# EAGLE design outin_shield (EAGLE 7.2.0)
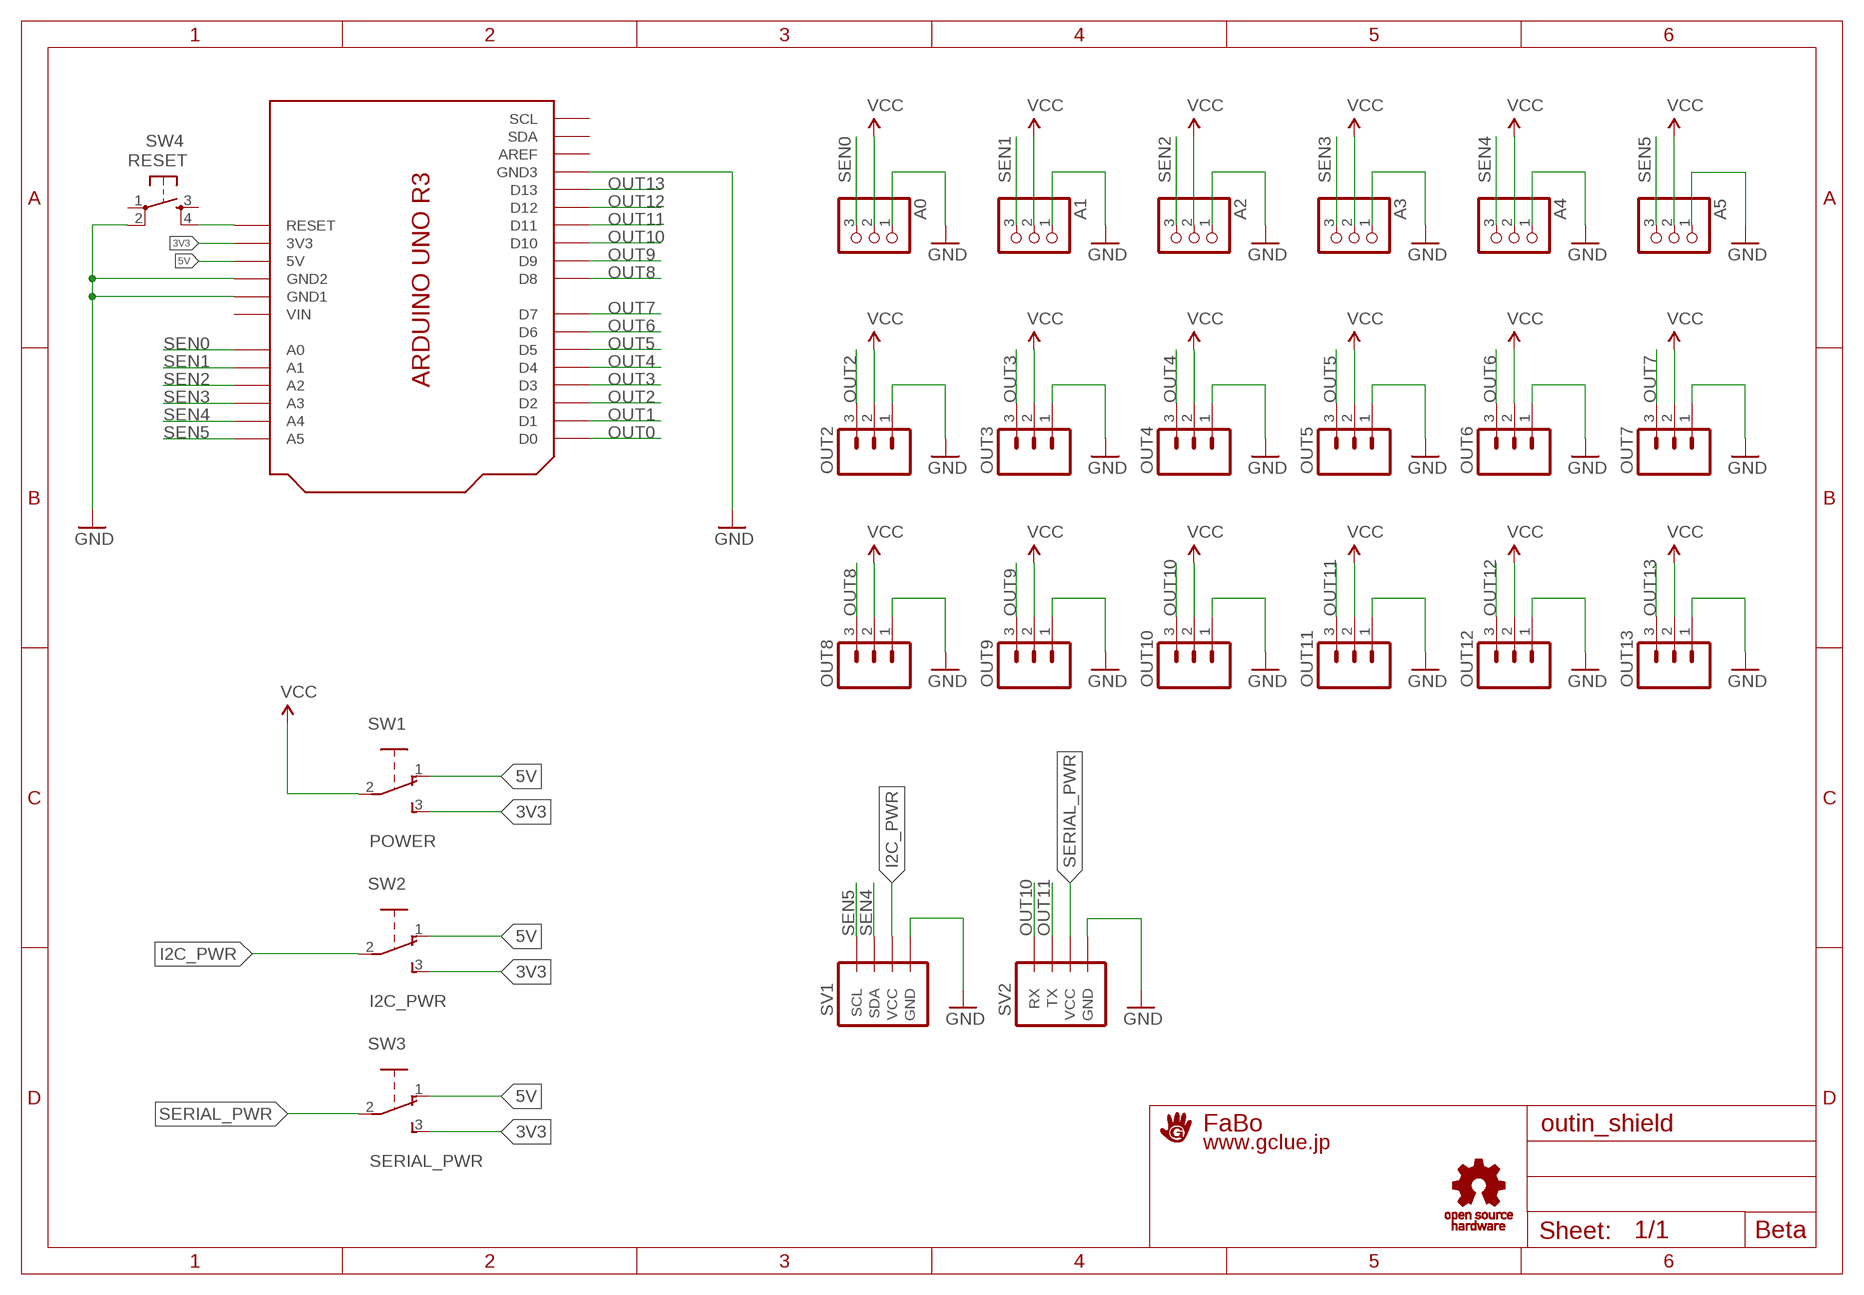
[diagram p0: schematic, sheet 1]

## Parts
A0  PINHD-1X3  [1X03]
A1  PINHD-1X3  [1X03]
A2  PINHD-1X3  [1X03]
A3  PINHD-1X3  [1X03]
A4  PINHD-1X3  [1X03]
A5  PINHD-1X3  [1X03]
OUT2  M03PTH  [1X03]
OUT3  M03PTH  [1X03]
OUT4  M03PTH  [1X03]
OUT5  M03PTH  [1X03]
OUT6  M03PTH  [1X03]
OUT7  M03PTH  [1X03]
OUT8  M03PTH  [1X03]
OUT9  M03PTH  [1X03]
OUT10  M03PTH  [1X03]
OUT11  M03PTH  [1X03]
OUT12  M03PTH  [1X03]
OUT13  M03PTH  [1X03]
SV1  BRICK_I2C_CONNECTOR  [BRICK_I2C_CONNECTOR]
SV2  BRICK_SERIAL_CONNECTOR  [BRICK_SERIAL_CONNECTOR]
SW1  POWER  SWITCH-SLIDE-EG1218  [EG1218]
SW2  I2C_PWR  SWITCH-SLIDE-EG1218  [EG1218]
SW3  SERIAL_PWR  SWITCH-SLIDE-EG1218  [EG1218]
SW4  RESET  TAC_SWITCHPTH  [TACTILE-PTH]
U1  OUTIN_SHIELD  [ARDUINO_UNO_R3_OUTIN]
U$2  LOGO_GCLUE-M  [LOGO_GCLUE_M]
U$3  LOGO_OSHW_T-M  [LOGO_OSHW_T_M]

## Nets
3V3 [POWER]: SW1.3 SW2.3 SW3.3 U1.3V3
5V [POWER]: SW1.1 SW2.1 SW3.1 U1.5V
GND [POWER]: A0.1 A1.1 A2.1 A3.1 A4.1 A5.1 OUT2.1 OUT3.1 OUT4.1 OUT5.1 OUT6.1 OUT7.1 OUT8.1 OUT9.1 OUT10.1 OUT11.1 OUT12.1 OUT13.1 SV1.GND SV2.GND SW4.2 U1.GND1 U1.GND2 U1.GND3
I2C_PWR [POWER]: SV1.VCC SW2.2
OUT0: U1.D0
OUT1: U1.D1
OUT2: OUT2.3 U1.D2
OUT3: OUT3.3 U1.D3
OUT4: OUT4.3 U1.D4
OUT5: OUT5.3 U1.D5
OUT6: OUT6.3 U1.D6
OUT7: OUT7.3 U1.D7
OUT8: OUT8.3 U1.D8
OUT9: OUT9.3 U1.D9
OUT10: OUT10.3 SV2.RX U1.D10
OUT11: OUT11.3 SV2.TX U1.D11
OUT12: OUT12.3 U1.D12
OUT13: OUT13.3 U1.D13
RESET: SW4.4 U1.RESET
SEN0: A0.3 U1.A0
SEN1: A1.3 U1.A1
SEN2: A2.3 U1.A2
SEN3: A3.3 U1.A3
SEN4: A4.3 SV1.SDA U1.A4
SEN5: A5.3 SV1.SCL U1.A5
SERIAL_PWR [POWER]: SV2.VCC SW3.2
VCC [POWER]: A0.2 A1.2 A2.2 A3.2 A4.2 A5.2 OUT2.2 OUT3.2 OUT4.2 OUT5.2 OUT6.2 OUT7.2 OUT8.2 OUT9.2 OUT10.2 OUT11.2 OUT12.2 OUT13.2 SW1.2
Unconnected: SW4.1 SW4.3 U1.AREF U1.SCL U1.SDA

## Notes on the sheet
- RESET
- Beta

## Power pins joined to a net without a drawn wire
VIN: U1.VIN

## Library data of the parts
A0 A1-A5 = adafruit:PINHD-1X3: PIN HEADER
OUT2-OUT13 = SparkFun:M03: Header 3 Standard 3-pin 0.1" header. Use with straight break away headers (SKU : PRT-00116), right angle break away headers (PRT-00553), swiss pins (PRT-00743), machine pins (PRT-00117), and female headers (PRT-00115). Molex polarized connector foot print use with SKU : PRT-08232 with associated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
SV1 = Gclue:BRICK_I2C_CONNECTOR: Brick Connector female for OUT/IN Shield
SV2 = Gclue:BRICK_SERIAL_CONNECTOR
SW1-SW3 = Gclue:SWITCH-SLIDE
SW4 = SparkFun-3-2-07:TAC_SWITCH: Momentary Switch Button commonly used for reset or general input. Spark Fun Electronics SKU : Comp-PBS
U1 = Gclue:OUTIN_SHIELD
U$2 = Gclue:LOGO_GCLUE
U$3 = Gclue:LOGO_OSHW_T

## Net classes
1 POWER: width 0.406 mm

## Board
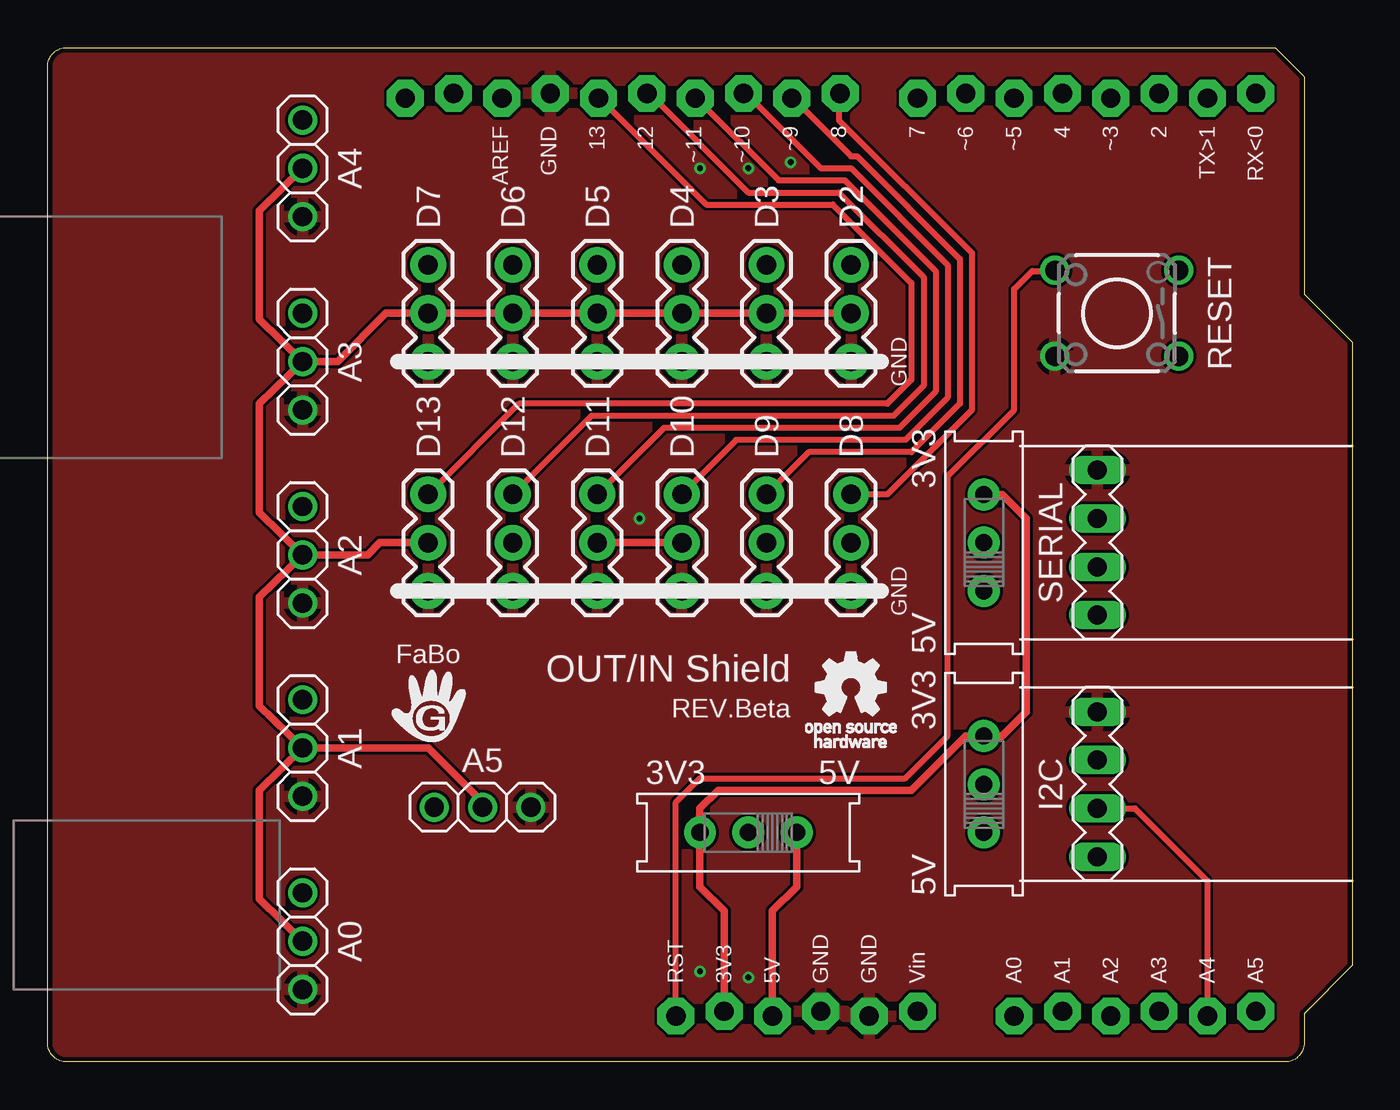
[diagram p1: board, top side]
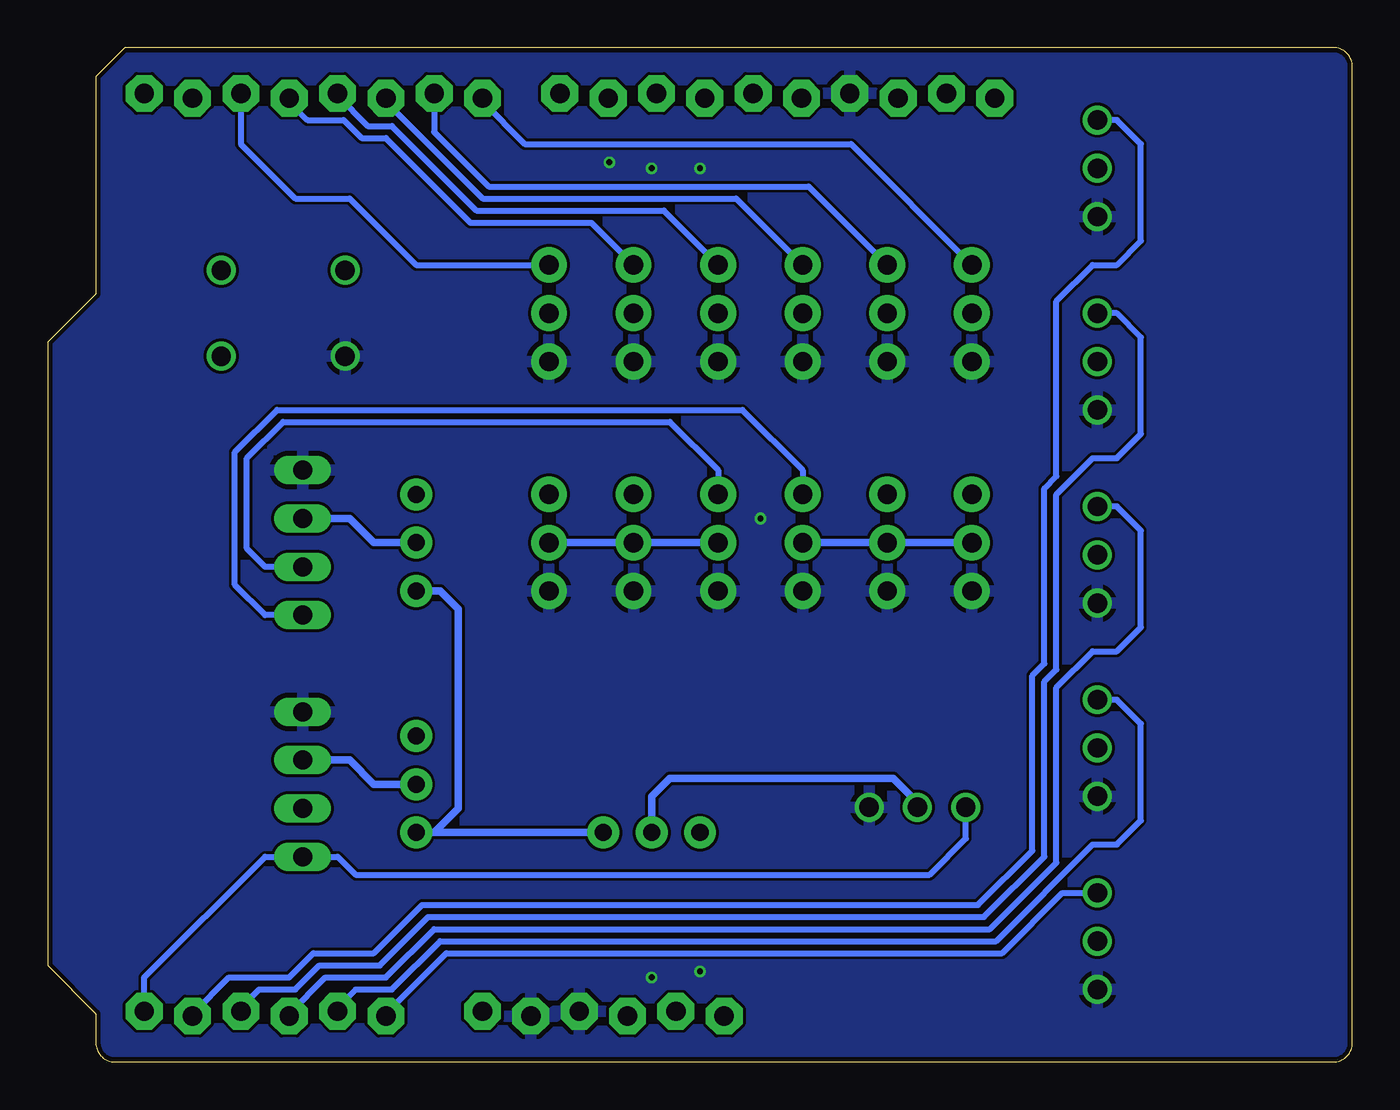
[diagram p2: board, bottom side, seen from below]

Size 68.58 x 53.34 mm. Coordinates in mm from the lower left corner, seen from the top.
Copper layers (1*16): Top 0.035mm / dielectric 1.5mm / Bottom 0.035mm
Design rules "Elecrow_2-layer_eagle_rule": minimum track width 6mil, minimum drill 12mil, track to track 6mil, track to pad 6mil, pad to pad 6mil, via to via 6mil, smd to smd 0mil, copper to edge 10mil, drill to drill 10mil, minimum pad ring 10mil, minimum via ring 6mil, stop-mask expansion 2mil, vias tented up to drill 100mil, thermal gap 10mil

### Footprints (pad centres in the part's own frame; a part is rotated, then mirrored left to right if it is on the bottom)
1X03 = drill 1.016: 1 -2.54,0; 2 0,0; 3 2.54,0
1X03' = drill 1.016 pad 1.88: 1 0,0; 2 2.54,0; 3 5.08,0
BRICK_I2C_CONNECTOR = drill 1 long: GND -3.81,0; SCL 3.81,0; SDA 1.27,0; VCC -1.27,0
BRICK_SERIAL_CONNECTOR = drill 1 long: GND -3.81,0; RX 1.27,0; TX 3.81,0; VCC -1.27,0
EG1218 = drill 0.9 pad 1.676: 1 -2.54,0; 2 0,0; 3 2.54,0
TACTILE-PTH = drill 1.016: 1 -3.251,2.261; 2 3.251,2.261; 3 -3.251,-2.261; 4 3.251,-2.261
ARDUINO_UNO_R3_OUTIN = drill 1.016 pad 1.93 octagon: 3V3 35.56,2.667; 5V 38.1,2.413; A0 50.8,2.413; A1 53.34,2.667; A2 55.88,2.413; A3 58.42,2.667; A4 60.96,2.413; A5 63.5,2.667; AREF 23.876,50.673; D0 63.5,50.927; D1 60.96,50.673; D2 58.42,50.927; D3 55.88,50.673; D4 53.34,50.927; D5 50.8,50.673; D6 48.26,50.927; D7 45.72,50.673; D8 41.656,50.927; D9 39.116,50.673; D10 36.576,50.927; D11 34.036,50.673; D12 31.496,50.927; D13 28.956,50.673; GND1 43.18,2.413; GND2 40.64,2.667; GND3 26.416,50.927; RESET 33.02,2.413; SCL 18.796,50.673; SDA 21.336,50.927; VIN 45.72,2.667

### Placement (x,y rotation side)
A0  13.4,6.35 90 top
A1  13.4,16.51 90 top
A2  13.4,26.67 90 top
A3  13.4,36.83 90 top
A4  13.4,46.99 90 top
A5  22.86,13.4 180 top
OUT2  [1X03']  42.23,36.83 90 top
OUT3  [1X03']  37.78,36.83 90 top
OUT4  [1X03']  33.34,36.83 90 top
OUT5  [1X03']  28.89,36.83 90 top
OUT6  [1X03']  24.45,36.83 90 top
OUT7  [1X03']  20,36.83 90 top
OUT8  [1X03']  42.23,24.77 90 top
OUT9  [1X03']  37.78,24.77 90 top
OUT10  [1X03']  33.34,24.77 90 top
OUT11  [1X03']  28.89,24.77 90 top
OUT12  [1X03']  24.45,24.77 90 top
OUT13  [1X03']  20,24.77 90 top
SV1  55.18,14.61 270 top
SV2  55.18,27.3 270 top
SW1  36.83,12.06 180 top
SW2  49.21,14.61 90 top
SW3  49.21,27.3 90 top
SW4  56.2,39.37 180 top
U1  0,0 0 top
U$2  20,18.73 0 top
U$3  42.23,19.68 0 top

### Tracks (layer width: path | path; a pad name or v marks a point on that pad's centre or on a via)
3V3
  Top 0.406: U1.3V3 35.56,7.94 34.29,9.21 SW1.3 34.29,13.34 35.24,14.29 45.4,14.29 48.26,17.14 SW2.3 50.16,17.14 51.44,18.41 51.44,28.57 50.16,29.84 SW3.3
5V
  Top 0.406: U1.5V 38.1,7.94 39.37,9.21 SW1.1
  Bottom 0.406: SW1.1 48.26,12.06 | SW2.1 48.26,12.06 | 48.26,12.06 46.99,13.34 46.99,23.81 47.94,24.77 SW3.1
GND  (via drill 0.3)
  other vias: 36.83,4.45 34.29,4.76 31.11,28.57 34.29,46.99 36.83,46.99 39.05,47.31
  pour Bottom: -7.3,54.29 69.53,54.29 69.53,-0.95 -7.3,-0.95
  pour Top: -7.3,54.29 69.53,54.29 69.53,-0.95 -7.3,-0.95
I2C_PWR
  Bottom 0.406: SW2.2 51.44,14.61 52.7,15.88 SV1.VCC
OUT2
  Bottom 0.305: U1.D2 58.42,48.26 55.56,45.4 52.7,45.4 49.21,41.91 OUT2.3
OUT3
  Bottom 0.305: U1.D3 55.88,50.48 54.93,49.53 53.02,49.53 52.07,48.58 50.8,48.58 46.35,44.13 40.01,44.13 OUT3.3
OUT4
  Bottom 0.305: U1.D4 53.34,50.8 51.75,49.21 50.48,49.21 46.04,44.77 36.2,44.77 OUT4.3
OUT5
  Bottom 0.305: U1.D5 50.8,50.48 45.72,45.4 32.38,45.4 OUT5.3
OUT6
  Bottom 0.305: U1.D6 48.26,48.9 45.4,46.04 28.57,46.04 OUT6.3
OUT7
  Bottom 0.305: U1.D7 45.72,50.48 43.5,48.26 26.35,48.26 OUT7.3
OUT8
  Top 0.305: U1.D8 41.59,50.8 41.59,49.53 48.58,42.55 48.58,34.29 44.13,29.84 OUT8.3
OUT9
  Top 0.305: U1.D9 39.37,50.48 42.23,47.62 42.55,47.62 47.94,42.23 47.94,34.61 45.4,32.07 40.01,32.07 OUT9.3
OUT10
  Top 0.305: U1.D10 36.83,50.8 40.64,46.99 42.23,46.99 47.31,41.91 47.31,34.92 45.09,32.7 36.2,32.7 OUT10.3
  Bottom 0.305: SV2.RX 57.15,26.04 58.1,26.99 58.1,31.75 56.2,33.66 35.88,33.66 33.34,31.11 OUT10.3
OUT11
  Top 0.305: U1.D11 34.29,50.48 38.42,46.35 41.91,46.35 46.67,41.59 46.67,35.24 44.77,33.34 32.38,33.34 OUT11.3
  Bottom 0.305: SV2.TX 57.15,23.5 58.74,25.08 58.74,32.07 56.52,34.29 32.07,34.29 28.89,31.11 OUT11.3
OUT12
  Top 0.305: U1.D12 31.75,50.8 36.83,45.72 41.59,45.72 46.04,41.27 46.04,35.56 44.45,33.97 28.57,33.97 OUT12.3
OUT13
  Top 0.305: U1.D13 29.21,50.48 34.61,45.09 41.27,45.09 45.4,40.96 45.4,35.88 44.13,34.61 24.77,34.61 OUT13.3
RESET
  Top 0.305: U1.RESET 33.02,13.65 34.29,14.92 45.09,14.92 47.31,17.14 47.31,30.8 50.8,34.29 50.8,40.64 51.75,41.59 52.7,41.59 SW4.4
SEN0
  Bottom 0.305: U1.A0 50.8,2.54 47.62,5.71 18.41,5.71 15.24,8.89 A0.3
SEN1
  Bottom 0.305: U1.A1 53.34,2.86 52.39,3.81 50.48,3.81 47.94,6.35 18.73,6.35 13.65,11.43 12.38,11.43 11.11,12.7 11.11,17.78 12.38,19.05 A1.3
SEN2
  Bottom 0.305: U1.A2 55.88,2.54 53.98,4.45 50.8,4.45 48.26,6.99 19.05,6.99 15.56,10.48 15.56,19.68 13.65,21.59 12.38,21.59 11.11,22.86 11.11,27.94 12.38,29.21 A2.3
SEN3
  Bottom 0.305: U1.A3 58.42,2.86 57.47,3.81 55.56,3.81 54.29,5.08 51.12,5.08 48.58,7.62 19.37,7.62 16.19,10.79 16.19,20 15.56,20.64 15.56,29.84 13.65,31.75 12.38,31.75 11.11,33.02 11.11,38.1 12.38,39.37 A3.3
SEN4
  Top 0.305: SV1.SDA 57.15,13.34 60.96,9.53 U1.A4
  Bottom 0.305: U1.A4 60.96,2.54 59.05,4.45 55.88,4.45 54.61,5.71 51.44,5.71 48.9,8.26 19.68,8.26 16.83,11.11 16.83,20.32 16.19,20.95 16.19,30.16 15.56,30.8 15.56,40.01 13.65,41.91 12.38,41.91 11.11,43.18 11.11,48.26 12.38,49.53 A4.3
SEN5
  Bottom 0.305: U1.A5 63.5,4.45 57.15,10.79 SV1.SCL 53.34,10.79 52.39,9.84 22.23,9.84 20.32,11.75 A5.3
SERIAL_PWR
  Bottom 0.406: SW3.2 51.44,27.3 52.7,28.57 SV2.VCC
VCC
  Top 0.406: A5.2 22.86,13.65 20,16.51 A1.2 | A1.2 11.11,14.29 11.11,8.57 A0.2 | A1.2 11.11,18.73 11.11,24.45 A2.2 | A2.2 11.11,28.89 11.11,34.61 A3.2 | A3.2 11.11,39.05 11.11,44.77 A4.2 | OUT11.2 OUT10.2 | OUT2.2 OUT3.2 OUT4.2 OUT5.2 OUT6.2 OUT7.2 17.78,39.37 15.24,36.83 A3.2 | A2.2 16.83,26.67 17.46,27.3 OUT13.2
  Bottom 0.406: SW1.2 36.83,13.97 35.88,14.92 24.13,14.92 22.86,13.65 A5.2 | OUT10.2 OUT9.2 OUT8.2 | OUT11.2 OUT12.2 OUT13.2

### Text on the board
tPlace: AREF | GND | 13 | 12 | ~11 | ~10 | ~9 | 8 | 7 | ~6 | ~5 | 4 | ~3 | 2 | TX>1 | RX<0 | A4 | D7 | D6 | D5 | D4 | D3 | D2 | RESET | A3 | GND | D13 | D12 | D11 | D10 | D9 | D8 | 3V3 | A2 | SERIAL | GND | 5V | FaBo | OUT/IN Shield | 3V3 | REV.Beta | A1 | A5 | 3V3 | 5V | I2C | 5V | A0 | RST | 3V3 | 5V | GND | GND | Vin | A0 | A1 | A2 | A3 | A4 | A5

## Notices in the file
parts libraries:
SparkFun: Licensing: CC v3.0 Share-Alike You are welcome to use this library for commercial purposes.
